(* Logix 5000 Routine export DNMon01Mapping; software revision 24.02 *)

TYPE AparianDNMGeneralStatus :
STRUCT
   Status : AparianDNMGeneralStatusFlags;
   ConfigCRC : INT;   // Configuration Checksum
   NodeStatus : AparianDNMNodeGeneralStatus[64];
   LiveCNHVoltage : REAL;   // Live CAN-H Voltage
   LiveCNLVoltage : REAL;   // Live CAN-L Voltage
   LivePowerVoltage : REAL;   // Live Power Voltage
   LiveShieldVoltage : REAL;   // Live Shield Voltage
   LiveCNHRaw : INT;   // Live CAN-H Raw
   LiveCNLRaw : INT;   // Live CAN-L Raw
   LivePowerRaw : INT;   // Live Power Raw
   LiveShieldRaw : INT;   // Live Shield Raw
   LiveCNHUncal : REAL;   // Live CAN-H Uncalibrated Voltage
   LiveCNLUncal : REAL;   // Live CAN-L Uncalibrated Voltage
   LivePowerUncal : REAL;   // Live Power Uncalibrated Voltage
   LiveShieldUncal : REAL;   // Live Shield Uncalibrated Voltage
   LastNodeProcessed : INT;   // Last Node Processed
   LastNodeTimeSinceProcessed : DINT;   // Time (ms) Since Last Node Processed
END_STRUCT
END_TYPE

TYPE AparianDNMNodeWarningAlarmStatus :
STRUCT
   DeviceNode : INT;   // Device Node Address
   SampleCount : DINT;   // Sample Count
   TimeSinceLastProcessed : DINT;   // Time (ms) since last processed
   PWRLowAlarm : AparianDNMChPwrStatus;   // Power Low Alarm
   PWRLowWarn : AparianDNMChPwrStatus;   // Power Low Warning
   PWRHighWarn : AparianDNMChPwrStatus;   // Power High Warning
   PWRHighAlarm : AparianDNMChPwrStatus;   // Power High Alarm
   PWRLowAlarmLatch : AparianDNMChPwrStatus;   // Power Low Alarm Latch
   PWRLowWarnLatch : AparianDNMChPwrStatus;   // Power Low Warning Latch
   PWRHighWarnLatch : AparianDNMChPwrStatus;   // Power High Warning Latch
   PWRHighAlarmLatch : AparianDNMChPwrStatus;   // Power High Alarm Latch
   SHDLowAlarm : AparianDNMChPwrStatus;   // Shield Low Alarm
   SHDLowWarn : AparianDNMChPwrStatus;   // Shield Low Warning
   SHDHighWarn : AparianDNMChPwrStatus;   // Shield High Warning
   SHDHighAlarm : AparianDNMChPwrStatus;   // Shield High Alarm
   SHDLowAlarmLatch : AparianDNMChPwrStatus;   // Shield Low Alarm Latch
   SHDLowWarnLatch : AparianDNMChPwrStatus;   // Shield Low Warning Latch
   SHDHighWarnLatch : AparianDNMChPwrStatus;   // Shield High Warning Latch
   SHDHighAlarmLatch : AparianDNMChPwrStatus;   // Shield High Alarm Latch
   CNLLowAlarm : AparianDNMChCommStatus;   // CAN-L Low Alarm
   CNLLowWarn : AparianDNMChCommStatus;   // CAN-L Low Warning
   CNLHighWarn : AparianDNMChCommStatus;   // CAN-L High Warning
   CNLHighAlarm : AparianDNMChCommStatus;   // CAN-L High Alarm
   CNLLowAlarmLatch : AparianDNMChCommStatus;   // CAN-L Low Alarm Latch
   CNLLowWarnLatch : AparianDNMChCommStatus;   // CAN-L Low Warning Latch
   CNLHighWarnLatch : AparianDNMChCommStatus;   // CAN-L High Warning Latch
   CNLHighAlarmLatch : AparianDNMChCommStatus;   // CAN-L High Alarm Latch
   CNHLowAlarm : AparianDNMChCommStatus;   // CAN-H Low Alarm
   CNHLowWarn : AparianDNMChCommStatus;   // CAN-H Low Warning
   CNHHighWarn : AparianDNMChCommStatus;   // CAN-H High Warning
   CNHHighAlarm : AparianDNMChCommStatus;   // CAN-H High Alarm
   CNHLowAlarmLatch : AparianDNMChCommStatus;   // CAN-H Low Alarm Latch
   CNHLowWarnLatch : AparianDNMChCommStatus;   // CAN-H Low Warning Latch
   CNHHighWarnLatch : AparianDNMChCommStatus;   // CAN-H High Warning Latch
   CNHHighAlarmLatch : AparianDNMChCommStatus;   // CAN-H High Alarm Latch
   CANLowAlarm : AparianDNMChCommStatus;   // CAN Low Alarm
   CANLowWarn : AparianDNMChCommStatus;   // CAN Low Warning
   CANHighWarn : AparianDNMChCommStatus;   // CAN High Warning
   CANHighAlarm : AparianDNMChCommStatus;   // CAN High Alarm
   CANLowAlarmLatch : AparianDNMChCommStatus;   // CAN Low Alarm Latch
   CANLowWarnLatch : AparianDNMChCommStatus;   // CAN Low Warning Latch
   CANHighWarnLatch : AparianDNMChCommStatus;   // CAN High Warning Latch
   CANHighAlarmLatch : AparianDNMChCommStatus;   // CAN High Alarm Latch
END_STRUCT
END_TYPE

TYPE AparianDNMChPwrStatus :
STRUCT
   VoltAll : BOOL;   // Voltage
   NoisePP : BOOL;   // Noise Peak-Peak
   NoiseRMSGen : BOOL;   // Noise RMS
END_STRUCT
END_TYPE

TYPE AparianDNMLiveMinMax :
STRUCT
   Latest : REAL;   // Most Recent Value
   Min : REAL;   // Minimum Value
   Max : REAL;   // Maximum Value
END_STRUCT
END_TYPE

TYPE AparianDNMNodeGeneralStatus :
STRUCT
   NodeActive : BOOL;   // Node Active (0=Inactive 1=Active)
   PowerAlarm : BOOL;   // Power Alarm (0=Ok 1=Alarm)
   PowerAlarmLatch : BOOL;   // Power Alarm Latch (0=Ok 1=AlarmLatch)
   PowerWarning : BOOL;   // Power Warning (0=Ok 1=Warning)
   PowerWarningLatch : BOOL;   // Power Warning Latch (0=Ok 1=WarningLatch)
   ShieldAlarm : BOOL;   // Shield Alarm (0=Ok 1=Alarm)
   ShieldAlarmLatch : BOOL;   // Shield Alarm Latch (0=Ok 1=AlarmLatch)
   ShieldWarning : BOOL;   // Shield Warning (0=Ok 1=Warning)
   ShieldWarningLatch : BOOL;   // Shield Warning Latch (0=Ok 1=WarningLatch)
   CANAlarm : BOOL;   // CAN Alarm (0=Ok 1=Alarm)
   CANAlarmLatch : BOOL;   // CAN Alarm Latch (0=Ok 1=AlarmLatch)
   CANWarning : BOOL;   // CAN Warning (0=Ok 1=Warning)
   CANWarningLatch : BOOL;   // CAN Warning Latch (0=Ok 1=WarningLatch)
   CNLAlarm : BOOL;   // CAN-L Alarm (0=Ok 1=Alarm)
   CNLAlarmLatch : BOOL;   // CAN-L Alarm Latch (0=Ok 1=AlarmLatch)
   CNLWarning : BOOL;   // CAN-L Warning (0=Ok 1=Warning)
   CNLWarningLatch : BOOL;   // CAN-L Warning Latch (0=Ok 1=WarningLatch)
   CNHAlarm : BOOL;   // CAN-H Alarm (0=Ok 1=Alarm)
   CNHAlarmLatch : BOOL;   // CAN-H Alarm Latch (0=Ok 1=AlarmLatch)
   CNHWarning : BOOL;   // CAN-H Warning (0=Ok 1=Warning)
   CNHWarningLatch : BOOL;   // CAN-H Warning Latch (0=Ok 1=WarningLatch)
END_STRUCT
END_TYPE

TYPE AparianDNMChCommStatus :
STRUCT
   VoltDom : BOOL;   // Dominant Voltage
   VoltRec : BOOL;   // Recessive Voltage
   VoltCM : BOOL;   // Common Mode Voltage
   RiseTime : BOOL;   // Rise Time
   FallTime : BOOL;   // Fall Time
   PosSlew : BOOL;   // Positive Slew Rate
   NegSlew : BOOL;   // Negative Slew Rate
   Overshoot : BOOL;   // Overshoot
   Undershoot : BOOL;   // Undershoot
   NoiseRMSDom : BOOL;   // Dominant Noise RMS
   NoiseRMSRec : BOOL;   // Recessive Noise RMS
   DroopDom : BOOL;   // Dominant Droop
   DroopRec : BOOL;   // Recessive Droop
END_STRUCT
END_TYPE

TYPE AparianDNMNodeLiveMinMax :
STRUCT
   DeviceNode : INT;   // Device Node Address
   PWRVoltAll : AparianDNMLiveMinMax;   // Power Voltage
   PWRNoisePP : AparianDNMLiveMinMax;   // Power Noise Peak-Peak
   PWRNoiseRMSGen : AparianDNMLiveMinMax;   // Power Noise RMS
   SHDVoltAll : AparianDNMLiveMinMax;   // Shield Voltage
   SHDNoisePP : AparianDNMLiveMinMax;   // Shield Noise Peak-Peak
   SHDNoiseRMSGen : AparianDNMLiveMinMax;   // Shield Noise RMS
   CNLVoltDom : AparianDNMLiveMinMax;   // CAN-L Dominant Voltage
   CNLVoltRec : AparianDNMLiveMinMax;   // CAN-L Recessive Voltage
   CNLPosSlew : AparianDNMLiveMinMax;   // CAN-L Positive Slew Rate
   CNLNegSlew : AparianDNMLiveMinMax;   // CAN-L Negative Slew Rate
   CNLOvershoot : AparianDNMLiveMinMax;   // CAN-L Overshoot
   CNLUndershoot : AparianDNMLiveMinMax;   // CAN-L Undershoot
   CNLNoiseRMSDom : AparianDNMLiveMinMax;   // CAN-L Dominant Noise RMS
   CNLNoiseRMSRec : AparianDNMLiveMinMax;   // CAN-L Recessive Noise RMS
   CNLDroopDom : AparianDNMLiveMinMax;   // CAN-L Dominant Droop
   CNLDroopRec : AparianDNMLiveMinMax;   // CAN-L Recessive Droop
   CNHVoltDom : AparianDNMLiveMinMax;   // CAN-H Dominant Voltage
   CNHVoltRec : AparianDNMLiveMinMax;   // CAN-H Recessive Voltage
   CNHPosSlew : AparianDNMLiveMinMax;   // CAN-H Positive Slew Rate
   CNHNegSlew : AparianDNMLiveMinMax;   // CAN-H Negative Slew Rate
   CNHOvershoot : AparianDNMLiveMinMax;   // CAN-H Overshoot
   CNHUndershoot : AparianDNMLiveMinMax;   // CAN-H Undershoot
   CNHNoiseRMSDom : AparianDNMLiveMinMax;   // CAN-H Dominant Noise RMS
   CNHNoiseRMSRec : AparianDNMLiveMinMax;   // CAN-H Recessive Noise RMS
   CNHDroopDom : AparianDNMLiveMinMax;   // CAN-H Dominant Droop
   CNHDroopRec : AparianDNMLiveMinMax;   // CAN-H Recessive Droop
   CANVoltDom : AparianDNMLiveMinMax;   // CAN Dominant Voltage
   CANVoltRec : AparianDNMLiveMinMax;   // CAN Recessive Voltage
   CANVoltCM : AparianDNMLiveMinMax;   // CAN Common Mode Voltage
   CANRiseTime : AparianDNMLiveMinMax;   // CAN Rise Time
   CANFallTime : AparianDNMLiveMinMax;   // CAN Fall Time
   CANPosSlew : AparianDNMLiveMinMax;   // CAN Positive Slew Rate
   CANNegSlew : AparianDNMLiveMinMax;   // CAN Negative Slew Rate
   CANOvershoot : AparianDNMLiveMinMax;   // CAN Overshoot
   CANUndershoot : AparianDNMLiveMinMax;   // CAN Undershoot
   CANNoiseRMSDom : AparianDNMLiveMinMax;   // CAN Dominant Noise RMS
   CANNoiseRMSRec : AparianDNMLiveMinMax;   // CAN Recessive Noise RMS
   CANDroopDom : AparianDNMLiveMinMax;   // CAN Dominant Droop
   CANDroopRec : AparianDNMLiveMinMax;   // CAN Recessive Droop
END_STRUCT
END_TYPE

TYPE AparianDNMGeneralStatusFlags :
STRUCT
   ConfigValid : BOOL;   // Configuration Valid (0=Invalid, 1=Valid)
   EIPOwned : BOOL;   // EtherNet/IP Ownership (0=Not Owned, 1=Owned)
   NTPOk : BOOL;   // Network Time Protocol (0=Invalid, 1= Ok)
   ControllerRun : BOOL;   // Controller Mode (0=Program, 1=Run)
   PowerCalibrationOk : BOOL;   // Power Channel Calibration (0=Fail, 1=Ok)
   ShieldCalibrationOk : BOOL;   // Shield Channel Calibration (0=Fail, 1=Ok)
   CANHCalibrationOk : BOOL;   // CAN-H Channel Calibration (0=Fail, 1=Ok)
   CANLCalibrationOk : BOOL;   // CAN-L Channel Calibration (0=Fail, 1=Ok)
END_STRUCT
END_TYPE

TYPE AparianDNMNodeWarningAlarmCounters :
STRUCT
   DeviceNode : INT;   // Device Node Address
   PWRVoltAllLowAlarm : DINT;   // Power Voltage Low Alarm Count
   PWRVoltAllLowWarn : DINT;   // Power Voltage Low Warning Count
   PWRVoltAllHighWarn : DINT;   // Power Voltage High Warning Count
   PWRVoltAllHighAlarm : DINT;   // Power Voltage High Alarm Count
   PWRNoisePPHighWarn : DINT;   // Power Noise Peak-Peak High Warning Count
   PWRNoisePPHighAlarm : DINT;   // Power Noise Peak-Peak High Alarm Count
   PWRNoiseRMSGenHighWarn : DINT;   // Power Noise RMS High Warning Count
   PWRNoiseRMSGenHighAlarm : DINT;   // Power Noise RMS High Alarm Count
   SHDVoltAllLowAlarm : DINT;   // Shield Voltage Low Alarm Count
   SHDVoltAllLowWarn : DINT;   // Shield Voltage Low Warning Count
   SHDVoltAllHighWarn : DINT;   // Shield Voltage High Warning Count
   SHDVoltAllHighAlarm : DINT;   // Shield Voltage High Alarm Count
   SHDNoisePPHighWarn : DINT;   // Shield Noise Peak-Peak High Warning Count
   SHDNoisePPHighAlarm : DINT;   // Shield Noise Peak-Peak High Alarm Count
   SHDNoiseRMSGenHighWarn : DINT;   // Shield Noise RMS High Warning Count
   SHDNoiseRMSGenHighAlarm : DINT;   // Shield Noise RMS High Alarm Count
   CNLVoltDomLowAlarm : DINT;   // CAN-L Dominant Voltage Low Alarm Count
   CNLVoltDomLowWarn : DINT;   // CAN-L Dominant Voltage Low Warning Count
   CNLVoltDomHighWarn : DINT;   // CAN-L Dominant Voltage High Warning Count
   CNLVoltDomHighAlarm : DINT;   // CAN-L Dominant Voltage High Alarm Count
   CNLVoltRecLowAlarm : DINT;   // CAN-L Recessive Voltage Low Alarm Count
   CNLVoltRecLowWarn : DINT;   // CAN-L Recessive Voltage Low Warning Count
   CNLVoltRecHighWarn : DINT;   // CAN-L Recessive Voltage High Warning Count
   CNLVoltRecHighAlarm : DINT;   // CAN-L Recessive Voltage High Alarm Count
   CNLPosSlewLowAlarm : DINT;   // CAN-L Positive Slew Rate Low Alarm Count
   CNLPosSlewLowWarn : DINT;   // CAN-L Positive Slew Rate Low Warning Count
   CNLPosSlewHighWarn : DINT;   // CAN-L Positive Slew Rate High Warning Count
   CNLPosSlewHighAlarm : DINT;   // CAN-L Positive Slew Rate High Alarm Count
   CNLNegSlewLowAlarm : DINT;   // CAN-L Negative Slew Rate Low Alarm Count
   CNLNegSlewLowWarn : DINT;   // CAN-L Negative Slew Rate Low Warning Count
   CNLNegSlewHighWarn : DINT;   // CAN-L Negative Slew Rate High Warning Count
   CNLNegSlewHighAlarm : DINT;   // CAN-L Negative Slew Rate High Alarm Count
   CNLOvershootHighWarn : DINT;   // CAN-L Overshoot High Warning Count
   CNLOvershootHighAlarm : DINT;   // CAN-L Overshoot High Alarm Count
   CNLUndershootHighWarn : DINT;   // CAN-L Undershoot High Warning Count
   CNLUndershootHighAlarm : DINT;   // CAN-L Undershoot High Alarm Count
   CNLNoiseRMSDomHighWarn : DINT;   // CAN-L Dominant Noise RMS High Warning Count
   CNLNoiseRMSDomHighAlarm : DINT;   // CAN-L Dominant Noise RMS High Alarm Count
   CNLNoiseRMSRecHighWarn : DINT;   // CAN-L Recessive Noise RMS High Warning Count
   CNLNoiseRMSRecHighAlarm : DINT;   // CAN-L Recessive Noise RMS High Alarm Count
   CNLDroopDomLowAlarm : DINT;   // CAN-L Dominant Droop Low Alarm Count
   CNLDroopDomLowWarn : DINT;   // CAN-L Dominant Droop Low Warning Count
   CNLDroopDomHighWarn : DINT;   // CAN-L Dominant Droop High Warning Count
   CNLDroopDomHighAlarm : DINT;   // CAN-L Dominant Droop High Alarm Count
   CNLDroopRecLowAlarm : DINT;   // CAN-L Recessive Droop Low Alarm Count
   CNLDroopRecLowWarn : DINT;   // CAN-L Recessive Droop Low Warning Count
   CNLDroopRecHighWarn : DINT;   // CAN-L Recessive Droop High Warning Count
   CNLDroopRecHighAlarm : DINT;   // CAN-L Recessive Droop High Alarm Count
   CNHVoltDomLowAlarm : DINT;   // CAN-H Dominant Voltage Low Alarm Count
   CNHVoltDomLowWarn : DINT;   // CAN-H Dominant Voltage Low Warning Count
   CNHVoltDomHighWarn : DINT;   // CAN-H Dominant Voltage High Warning Count
   CNHVoltDomHighAlarm : DINT;   // CAN-H Dominant Voltage High Alarm Count
   CNHVoltRecLowAlarm : DINT;   // CAN-H Recessive Voltage Low Alarm Count
   CNHVoltRecLowWarn : DINT;   // CAN-H Recessive Voltage Low Warning Count
   CNHVoltRecHighWarn : DINT;   // CAN-H Recessive Voltage High Warning Count
   CNHVoltRecHighAlarm : DINT;   // CAN-H Recessive Voltage High Alarm Count
   CNHPosSlewLowAlarm : DINT;   // CAN-H Positive Slew Rate Low Alarm Count
   CNHPosSlewLowWarn : DINT;   // CAN-H Positive Slew Rate Low Warning Count
   CNHPosSlewHighWarn : DINT;   // CAN-H Positive Slew Rate High Warning Count
   CNHPosSlewHighAlarm : DINT;   // CAN-H Positive Slew Rate High Alarm Count
   CNHNegSlewLowAlarm : DINT;   // CAN-H Negative Slew Rate Low Alarm Count
   CNHNegSlewLowWarn : DINT;   // CAN-H Negative Slew Rate Low Warning Count
   CNHNegSlewHighWarn : DINT;   // CAN-H Negative Slew Rate High Warning Count
   CNHNegSlewHighAlarm : DINT;   // CAN-H Negative Slew Rate High Alarm Count
   CNHOvershootHighWarn : DINT;   // CAN-H Overshoot High Warning Count
   CNHOvershootHighAlarm : DINT;   // CAN-H Overshoot High Alarm Count
   CNHUndershootHighWarn : DINT;   // CAN-H Undershoot High Warning Count
   CNHUndershootHighAlarm : DINT;   // CAN-H Undershoot High Alarm Count
   CNHNoiseRMSDomHighWarn : DINT;   // CAN-H Dominant Noise RMS High Warning Count
   CNHNoiseRMSDomHighAlarm : DINT;   // CAN-H Dominant Noise RMS High Alarm Count
   CNHNoiseRMSRecHighWarn : DINT;   // CAN-H Recessive Noise RMS High Warning Count
   CNHNoiseRMSRecHighAlarm : DINT;   // CAN-H Recessive Noise RMS High Alarm Count
   CNHDroopDomLowAlarm : DINT;   // CAN-H Dominant Droop Low Alarm Count
   CNHDroopDomLowWarn : DINT;   // CAN-H Dominant Droop Low Warning Count
   CNHDroopDomHighWarn : DINT;   // CAN-H Dominant Droop High Warning Count
   CNHDroopDomHighAlarm : DINT;   // CAN-H Dominant Droop High Alarm Count
   CNHDroopRecLowAlarm : DINT;   // CAN-H Recessive Droop Low Alarm Count
   CNHDroopRecLowWarn : DINT;   // CAN-H Recessive Droop Low Warning Count
   CNHDroopRecHighWarn : DINT;   // CAN-H Recessive Droop High Warning Count
   CNHDroopRecHighAlarm : DINT;   // CAN-H Recessive Droop High Alarm Count
   CANVoltDomHighWarn : DINT;   // CAN Dominant Voltage High Warning Count
   CANVoltDomHighAlarm : DINT;   // CAN Dominant Voltage High Alarm Count
   CANVoltRecLowAlarm : DINT;   // CAN Recessive Voltage Low Alarm Count
   CANVoltRecLowWarn : DINT;   // CAN Recessive Voltage Low Warning Count
   CANVoltCMLowAlarm : DINT;   // CAN Common Mode Voltage Low Alarm Count
   CANVoltCMLowWarn : DINT;   // CAN Common Mode Voltage Low Warning Count
   CANVoltCMHighWarn : DINT;   // CAN Common Mode Voltage High Warning Count
   CANVoltCMHighAlarm : DINT;   // CAN Common Mode Voltage High Alarm Count
   CANRiseTimeLowAlarm : DINT;   // CAN Rise Time Low Alarm Count
   CANRiseTimeLowWarn : DINT;   // CAN Rise Time Low Warning Count
   CANRiseTimeHighWarn : DINT;   // CAN Rise Time High Warning Count
   CANRiseTimeHighAlarm : DINT;   // CAN Rise Time High Alarm Count
   CANFallTimeLowAlarm : DINT;   // CAN Fall Time Low Alarm Count
   CANFallTimeLowWarn : DINT;   // CAN Fall Time Low Warning Count
   CANFallTimeHighWarn : DINT;   // CAN Fall Time High Warning Count
   CANFallTimeHighAlarm : DINT;   // CAN Fall Time High Alarm Count
   CANPosSlewLowAlarm : DINT;   // CAN Positive Slew Rate Low Alarm Count
   CANPosSlewLowWarn : DINT;   // CAN Positive Slew Rate Low Warning Count
   CANPosSlewHighWarn : DINT;   // CAN Positive Slew Rate High Warning Count
   CANPosSlewHighAlarm : DINT;   // CAN Positive Slew Rate High Alarm Count
   CANNegSlewLowAlarm : DINT;   // CAN Negative Slew Rate Low Alarm Count
   CANNegSlewLowWarn : DINT;   // CAN Negative Slew Rate Low Warning Count
   CANNegSlewHighWarn : DINT;   // CAN Negative Slew Rate High Warning Count
   CANNegSlewHighAlarm : DINT;   // CAN Negative Slew Rate High Alarm Count
   CANOvershootHighWarn : DINT;   // CAN Overshoot High Warning Count
   CANOvershootHighAlarm : DINT;   // CAN Overshoot High Alarm Count
   CANUndershootHighWarn : DINT;   // CAN Undershoot High Warning Count
   CANUndershootHighAlarm : DINT;   // CAN Undershoot High Alarm Count
   CANNoiseRMSDomHighWarn : DINT;   // CAN Dominant Noise RMS High Warning Count
   CANNoiseRMSDomHighAlarm : DINT;   // CAN Dominant Noise RMS High Alarm Count
   CANNoiseRMSRecHighWarn : DINT;   // CAN Recessive Noise RMS High Warning Count
   CANNoiseRMSRecHighAlarm : DINT;   // CAN Recessive Noise RMS High Alarm Count
   CANDroopDomLowAlarm : DINT;   // CAN Dominant Droop Low Alarm Count
   CANDroopDomLowWarn : DINT;   // CAN Dominant Droop Low Warning Count
   CANDroopDomHighWarn : DINT;   // CAN Dominant Droop High Warning Count
   CANDroopDomHighAlarm : DINT;   // CAN Dominant Droop High Alarm Count
   CANDroopRecLowAlarm : DINT;   // CAN Recessive Droop Low Alarm Count
   CANDroopRecLowWarn : DINT;   // CAN Recessive Droop Low Warning Count
   CANDroopRecHighWarn : DINT;   // CAN Recessive Droop High Warning Count
   CANDroopRecHighAlarm : DINT;   // CAN Recessive Droop High Alarm Count
END_STRUCT
END_TYPE

ADD_ON_INSTRUCTION AparianDNMMap   (* revision 1.0, vendor Aparian *)
VAR_OUTPUT
   ConnectedOk : BOOL; {access Read Only, visible}
END_VAR
VAR_INPUT
   MuxNodeMax : INT := 63; {visible}
   MuxRate : DINT := 300; {visible}
   ResetStatistics : BOOL; {visible}
END_VAR
VAR_OUTPUT
   LastNodeProcessed : INT; {visible}
   MuxNode : INT; {access Read Only, visible}
END_VAR
VAR_INPUT
   ConnectionFaulted : BOOL; {required}
END_VAR
VAR_IN_OUT
   RawInput1 : SINT[500]; {required}
   RawInput2 : SINT[500]; {required}
   RawInput3 : SINT[500]; {required}
   RawInput4 : SINT[500]; {required}
   RawOutput1 : SINT[496]; {required}
   GeneralStatus : AparianDNMGeneralStatus; {required}
   NodeMinMax : AparianDNMNodeLiveMinMax[64]; {required}
   NodeAWCounters : AparianDNMNodeWarningAlarmCounters[64]; {required}
   NodeAWStatus : AparianDNMNodeWarningAlarmStatus[64]; {required}
END_VAR
VAR
   MuxTimer : TIMER; {access None}
   OwnedOk : BOOL; {access None}
   InMuxNode4 : INT; {access None}
   InMuxNode3 : INT; {access None}
   InMuxNode2 : INT; {access None}
   CmdMuxNode : DINT; {access None}
   ControlWord : DINT; {access None}
END_VAR

ROUTINE Logic   (* ladder *)
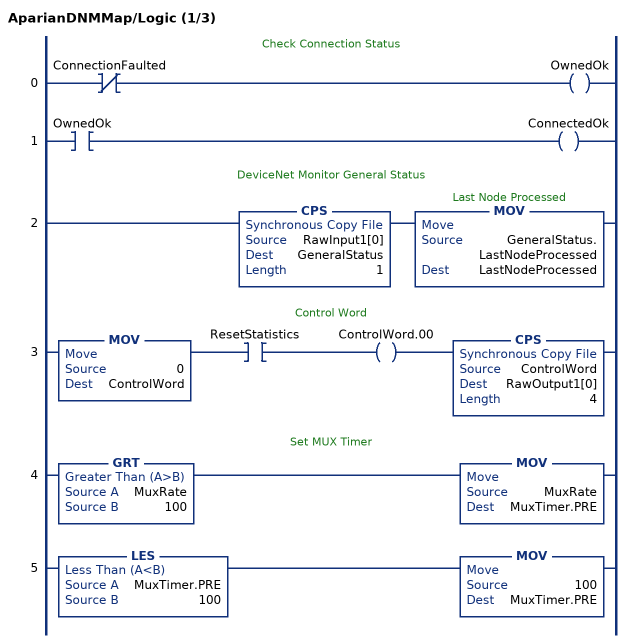
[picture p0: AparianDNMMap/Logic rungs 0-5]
   // Check Connection Status
   0: XIO(ConnectionFaulted)OTE(OwnedOk);
   1: XIC(OwnedOk)OTE(ConnectedOk);
   // DeviceNet Monitor General Status
   2: CPS(RawInput1[0],GeneralStatus,1)MOV(GeneralStatus.LastNodeProcessed,LastNodeProcessed);
   // Control Word
   3: MOV(0,ControlWord)XIC(ResetStatistics)OTE(ControlWord.00)CPS(ControlWord,RawOutput1[0],4);
   // Set MUX Timer
   4: GRT(MuxRate,100)MOV(MuxRate,MuxTimer.PRE);
   5: LES(MuxTimer.PRE,100)MOV(100,MuxTimer.PRE);
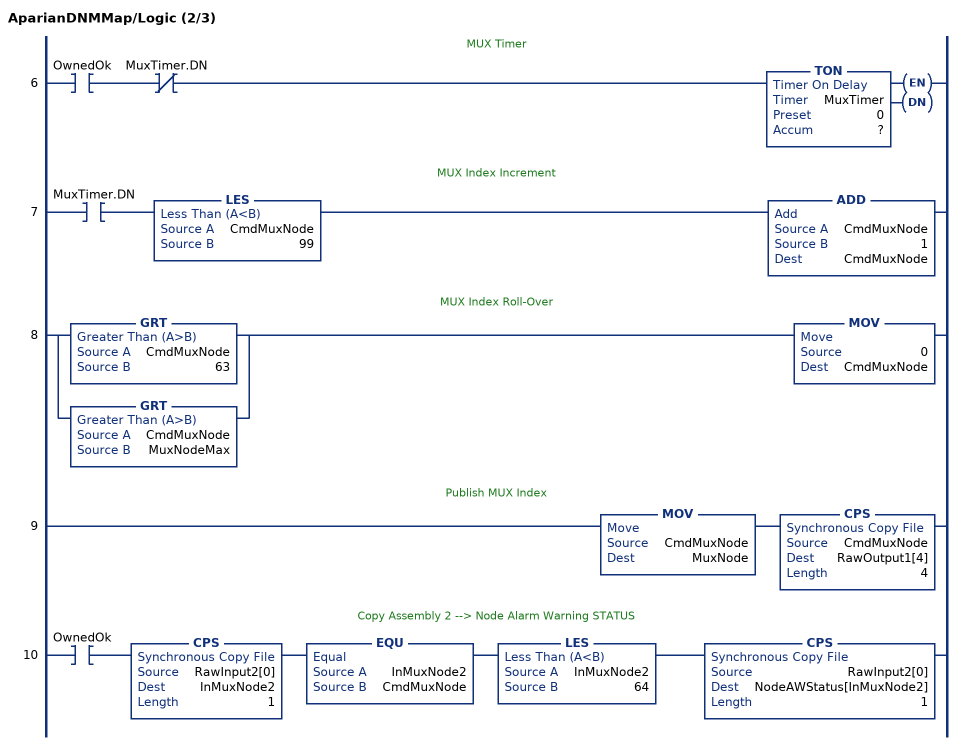
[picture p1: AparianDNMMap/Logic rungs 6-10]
   // MUX Timer
   6: XIC(OwnedOk)XIO(MuxTimer.DN)TON(MuxTimer,?,?);
   // MUX Index Increment
   7: XIC(MuxTimer.DN)LES(CmdMuxNode,99)ADD(CmdMuxNode,1,CmdMuxNode);
   // MUX Index Roll-Over
   8: [GRT(CmdMuxNode,63) ,GRT(CmdMuxNode,MuxNodeMax) ]MOV(0,CmdMuxNode);
   // Publish MUX Index
   9: MOV(CmdMuxNode,MuxNode)CPS(CmdMuxNode,RawOutput1[4],4);
   // Copy Assembly 2 --> Node Alarm Warning STATUS
   10: XIC(OwnedOk)CPS(RawInput2[0],InMuxNode2,1)EQU(InMuxNode2,CmdMuxNode)LES(InMuxNode2,64)CPS(RawInput2[0],NodeAWStatus[InMuxNode2],1);
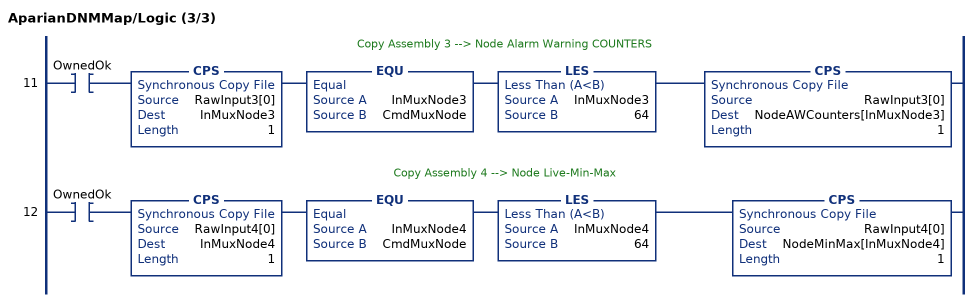
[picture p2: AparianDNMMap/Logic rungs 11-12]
   // Copy Assembly 3 --> Node Alarm Warning COUNTERS
   11: XIC(OwnedOk)CPS(RawInput3[0],InMuxNode3,1)EQU(InMuxNode3,CmdMuxNode)LES(InMuxNode3,64)CPS(RawInput3[0],NodeAWCounters[InMuxNode3],1);
   // Copy Assembly 4 --> Node Live-Min-Max
   12: XIC(OwnedOk)CPS(RawInput4[0],InMuxNode4,1)EQU(InMuxNode4,CmdMuxNode)LES(InMuxNode4,64)CPS(RawInput4[0],NodeMinMax[InMuxNode4],1);
END_ROUTINE
END_ADD_ON_INSTRUCTION

VAR_GLOBAL   (* controller tags *)
   DNMonMap01 : AparianDNMMap := (ConnectedOk := 1, MuxNodeMax := 18, MuxRate := 1100, LastNodeProcessed := 18, MuxNode := 9);
   DNM01NodeAWCounters : AparianDNMNodeWarningAlarmCounters[64];
   DNM01NodeAWStatus : AparianDNMNodeWarningAlarmStatus[64];
   DNM01GeneralStatus : AparianDNMGeneralStatus;
   DNM01NodeMinMax : AparianDNMNodeLiveMinMax[64];
END_VAR

PROGRAM MainProgram

ROUTINE DNMon01Mapping   (* ladder *)
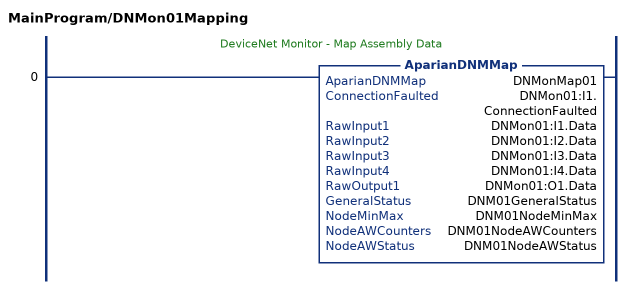
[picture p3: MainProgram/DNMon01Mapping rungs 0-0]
   // DeviceNet Monitor - Map Assembly Data
   0: AparianDNMMap(DNMonMap01,DNMon01:I1.ConnectionFaulted,DNMon01:I1.Data,DNMon01:I2.Data,DNMon01:I3.Data,DNMon01:I4.Data,DNMon01:O1.Data,DNM01GeneralStatus,DNM01NodeMinMax,DNM01NodeAWCounters,DNM01NodeAWStatus);
END_ROUTINE
END_PROGRAM
